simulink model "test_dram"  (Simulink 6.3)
settings: Solver=ode45  StartTime=0.0  StopTime=1024  RelTol=1e-3
undefined symbols (not defined in the file or in its folder): netlist
libraries: xbsIndex_r4 x9, simulink x5, adlibrary2 x2, dram_cosim_lib x1

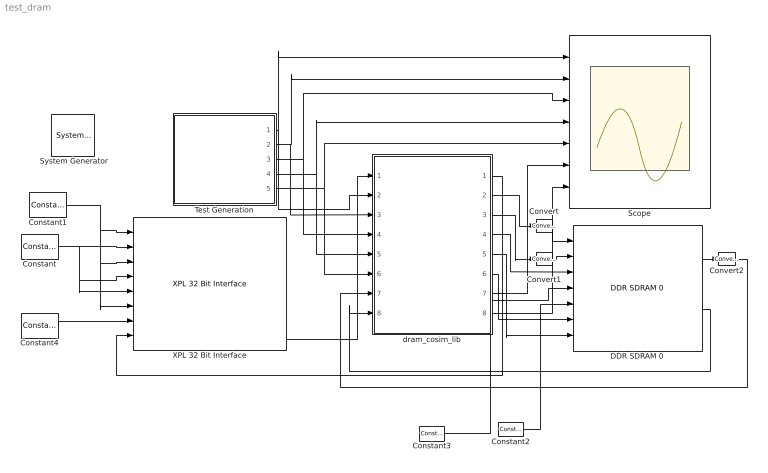
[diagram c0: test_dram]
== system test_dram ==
  " System Generator" : xbsIndex_r4/ System Generator  Tag=genX  xilinxfamily=Virtex2P  part=xc2vp70  speed=-5  package=ff1704  synthesis_tool=XST  directory=./netlist  testbench=off  simulink_period=1  sysclk_period=10  incr_netlist=off  trim_vbits=Everywhere in SubSystem  dbl_ovrd=According to Block Masks  core_generation=According to Block Masks  run_coregen=off  deprecated_control=off  eval_field=0  block_type=sysgen
  Constant : xbsIndex_r4/Constant  arith_type=Boolean  const=0  n_bits=16  bin_pt=14  explicit_period=on  period=1  equ=P=C  opselect=C  inp2=PCIN>>17  opr=+  inp1=P  carry=CIN  dbl_ovrd=off  block_type=constant
  Constant1 : xbsIndex_r4/Constant  arith_type=Unsigned  const=0  n_bits=32  bin_pt=0  explicit_period=on  period=1  equ=P=C  opselect=C  inp2=PCIN>>17  opr=+  inp1=P  carry=CIN  dbl_ovrd=off  block_type=constant
  Constant2 : xbsIndex_r4/Constant  arith_type=Unsigned  const=0  n_bits=4  bin_pt=0  explicit_period=on  period=1  equ=P=C  opselect=C  inp2=PCIN>>17  opr=+  inp1=P  carry=CIN  dbl_ovrd=off  block_type=constant
  Constant3 : xbsIndex_r4/Constant  arith_type=Unsigned  const=0  n_bits=15  bin_pt=0  explicit_period=on  period=1  equ=P=C  opselect=C  inp2=PCIN>>17  opr=+  inp1=P  carry=CIN  dbl_ovrd=off  block_type=constant
  Constant4 : xbsIndex_r4/Constant  arith_type=Unsigned  const=0  n_bits=66  bin_pt=0  explicit_period=on  period=1  equ=P=C  opselect=C  inp2=PCIN>>17  opr=+  inp1=P  carry=CIN  dbl_ovrd=off  block_type=constant
  Convert : xbsIndex_r4/Convert  arith_type=Unsigned  n_bits=32  bin_pt=0  quantization=Truncate  overflow=Wrap  latency=0  dbl_ovrd=off  pipeline=off  block_type=convert
  Convert1 : xbsIndex_r4/Convert  arith_type=Unsigned  n_bits=11  bin_pt=0  quantization=Truncate  overflow=Wrap  latency=0  dbl_ovrd=off  pipeline=off  block_type=convert
  Convert2 : xbsIndex_r4/Convert  arith_type=Unsigned  n_bits=16  bin_pt=0  quantization=Truncate  overflow=Wrap  latency=0  dbl_ovrd=off  pipeline=off  block_type=convert
  DDR SDRAM 0 : adlibrary2/ADP-XPI/DDR SDRAM 0  memsize=1
  Scope : Scope  NumInputPorts=7
  Test Generation : Subsystem
  XPL 32 Bit Interface : adlibrary2/ADM-XPL/XPL 32 Bit Interface  program='load myprogram.txt'  clock_ratio=1.5
  dram_cosim_lib : Subsystem  Tag=configX  BlockChoice=dram_cosim_lib_sim
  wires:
  Constant/1 -> XPL 32 Bit Interface/5, XPL 32 Bit Interface/4, XPL 32 Bit Interface/2
  Constant1/1 -> XPL 32 Bit Interface/6, XPL 32 Bit Interface/3, XPL 32 Bit Interface/1
  Test Generation/1(d) -> Scope/1, dram_cosim_lib/2(d_sl)
  Test Generation/2(a) -> Scope/2, dram_cosim_lib/3(a_sl)
  Test Generation/3(w) -> Scope/3, dram_cosim_lib/4(w_sl)
  Test Generation/4(dw) -> Scope/4, dram_cosim_lib/5(dw_sl)
  Test Generation/5(dr) -> Scope/5, dram_cosim_lib/6(dr_sl)
  XPL 32 Bit Interface/11 -> dram_cosim_lib/1(debug_in)
  dram_cosim_lib/1(debug_out) -> XPL 32 Bit Interface/8
  DDR SDRAM 0/2 -> dram_cosim_lib/8(busy_sg)
  DDR SDRAM 0/1 -> Convert2/1
  dram_cosim_lib/2(d_sg) -> Convert/1
  dram_cosim_lib/3(a_sg) -> Convert1/1
  dram_cosim_lib/4(w_sg) -> DDR SDRAM 0/3
  dram_cosim_lib/5(dw_sg) -> DDR SDRAM 0/7
  dram_cosim_lib/6(dr_sg) -> DDR SDRAM 0/6
  dram_cosim_lib/7(q_sl) -> Scope/6
  dram_cosim_lib/8(busy_sl) -> Scope/7
  Convert/1 -> DDR SDRAM 0/1
  Convert1/1 -> DDR SDRAM 0/2
  Constant2/1 -> DDR SDRAM 0/5
  Constant3/1 -> DDR SDRAM 0/4
  Convert2/1 -> dram_cosim_lib/7(q_sg)
  Constant4/1 -> XPL 32 Bit Interface/7

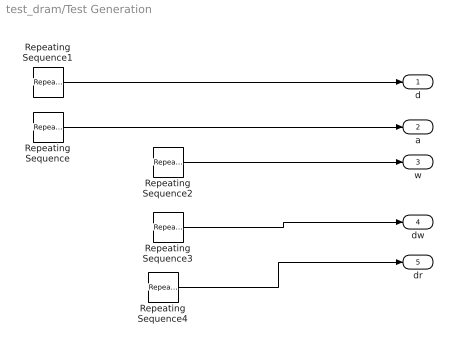
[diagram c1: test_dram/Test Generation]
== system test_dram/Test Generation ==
  Repeating Sequence : simulink/Sources/Repeating Sequence  rep_seq_t=[1:64]  rep_seq_y=[0:63]
  Repeating Sequence1 : simulink/Sources/Repeating Sequence  rep_seq_t=[1:1024]  rep_seq_y=[0:1023]
  Repeating Sequence2 : simulink/Sources/Repeating Sequence  rep_seq_t=[1:256]  rep_seq_y=[ones(1,64) zeros(1,3*64)]
  Repeating Sequence3 : simulink/Sources/Repeating Sequence  rep_seq_t=[1:1024]  rep_seq_y=[zeros(1,64) 1 zeros(1,15*64-1)]
  Repeating Sequence4 : simulink/Sources/Repeating Sequence  rep_seq_t=[1:1024]  rep_seq_y=[zeros(1,64*10) 1 zeros(1,6*64-1)]
  d : Outport
  a : Outport  Port=2
  w : Outport  Port=3
  dw : Outport  Port=4
  dr : Outport  Port=5
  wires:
  Repeating Sequence/1 -> a/1
  Repeating Sequence2/1 -> w/1
  Repeating Sequence1/1 -> d/1
  Repeating Sequence3/1 -> dw/1
  Repeating Sequence4/1 -> dr/1

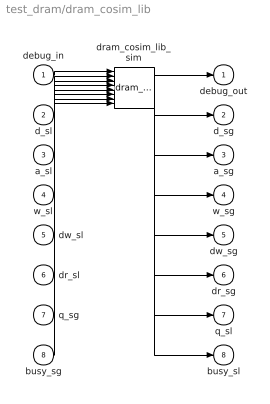
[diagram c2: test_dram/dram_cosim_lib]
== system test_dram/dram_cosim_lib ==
  debug_in : Inport
  d_sl : Inport  Port=2
  a_sl : Inport  Port=3
  w_sl : Inport  Port=4
  dw_sl : Inport  Port=5
  dr_sl : Inport  Port=6
  q_sg : Inport  Port=7
  busy_sg : Inport  Port=8
  dram_cosim_lib_sim : dram_cosim_lib/dram_cosim_lib_sim
  debug_out : Outport
  d_sg : Outport  Port=2
  a_sg : Outport  Port=3
  w_sg : Outport  Port=4
  dw_sg : Outport  Port=5
  dr_sg : Outport  Port=6
  q_sl : Outport  Port=7
  busy_sl : Outport  Port=8
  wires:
  debug_in/1 -> dram_cosim_lib_sim/1
  d_sl/1 -> dram_cosim_lib_sim/2
  a_sl/1 -> dram_cosim_lib_sim/3
  w_sl/1 -> dram_cosim_lib_sim/4
  dw_sl/1 -> dram_cosim_lib_sim/5
  dr_sl/1 -> dram_cosim_lib_sim/6
  q_sg/1 -> dram_cosim_lib_sim/7
  busy_sg/1 -> dram_cosim_lib_sim/8
  dram_cosim_lib_sim/1 -> debug_out/1
  dram_cosim_lib_sim/2 -> d_sg/1
  dram_cosim_lib_sim/3 -> a_sg/1
  dram_cosim_lib_sim/4 -> w_sg/1
  dram_cosim_lib_sim/5 -> dw_sg/1
  dram_cosim_lib_sim/6 -> dr_sg/1
  dram_cosim_lib_sim/7 -> q_sl/1
  dram_cosim_lib_sim/8 -> busy_sl/1
